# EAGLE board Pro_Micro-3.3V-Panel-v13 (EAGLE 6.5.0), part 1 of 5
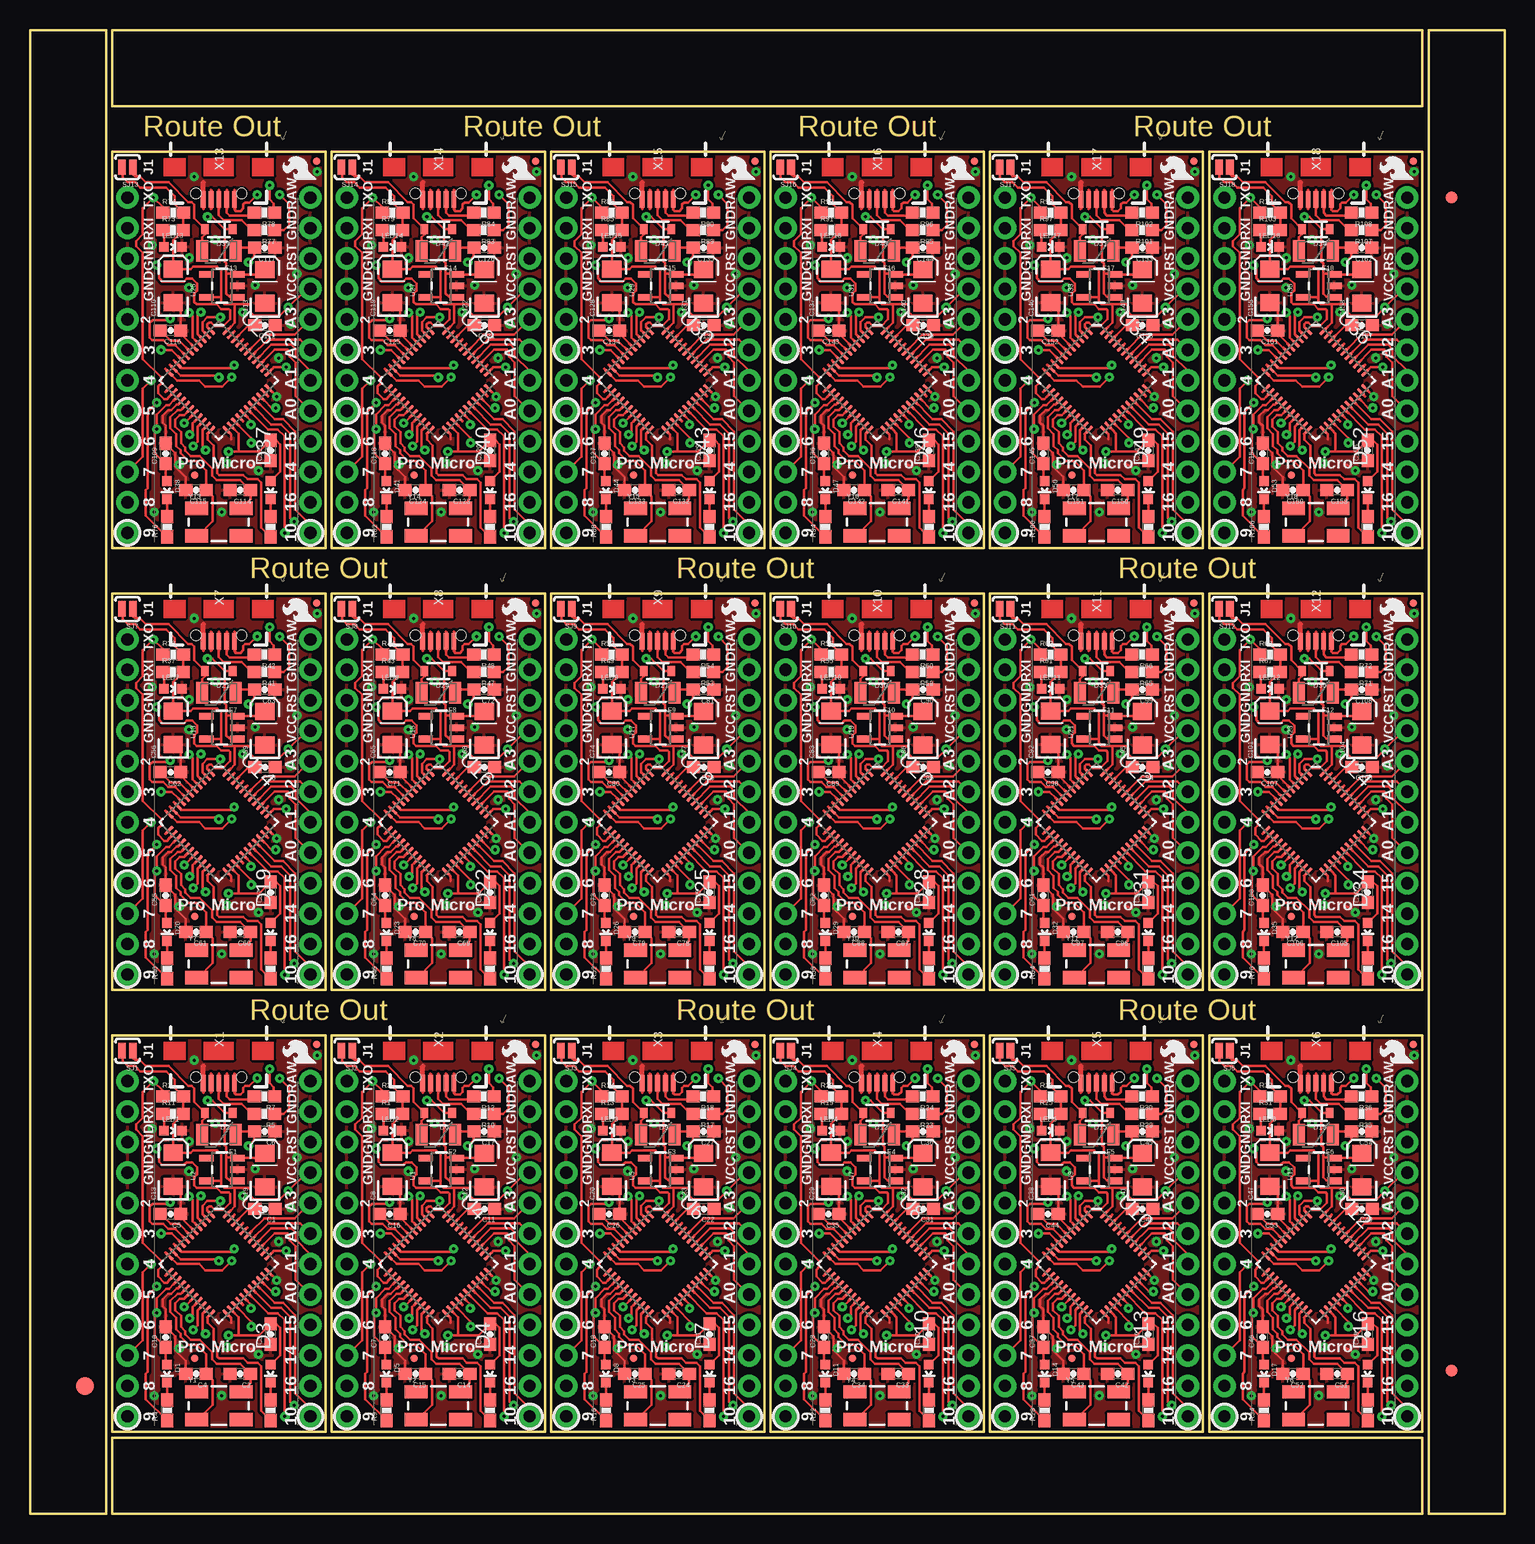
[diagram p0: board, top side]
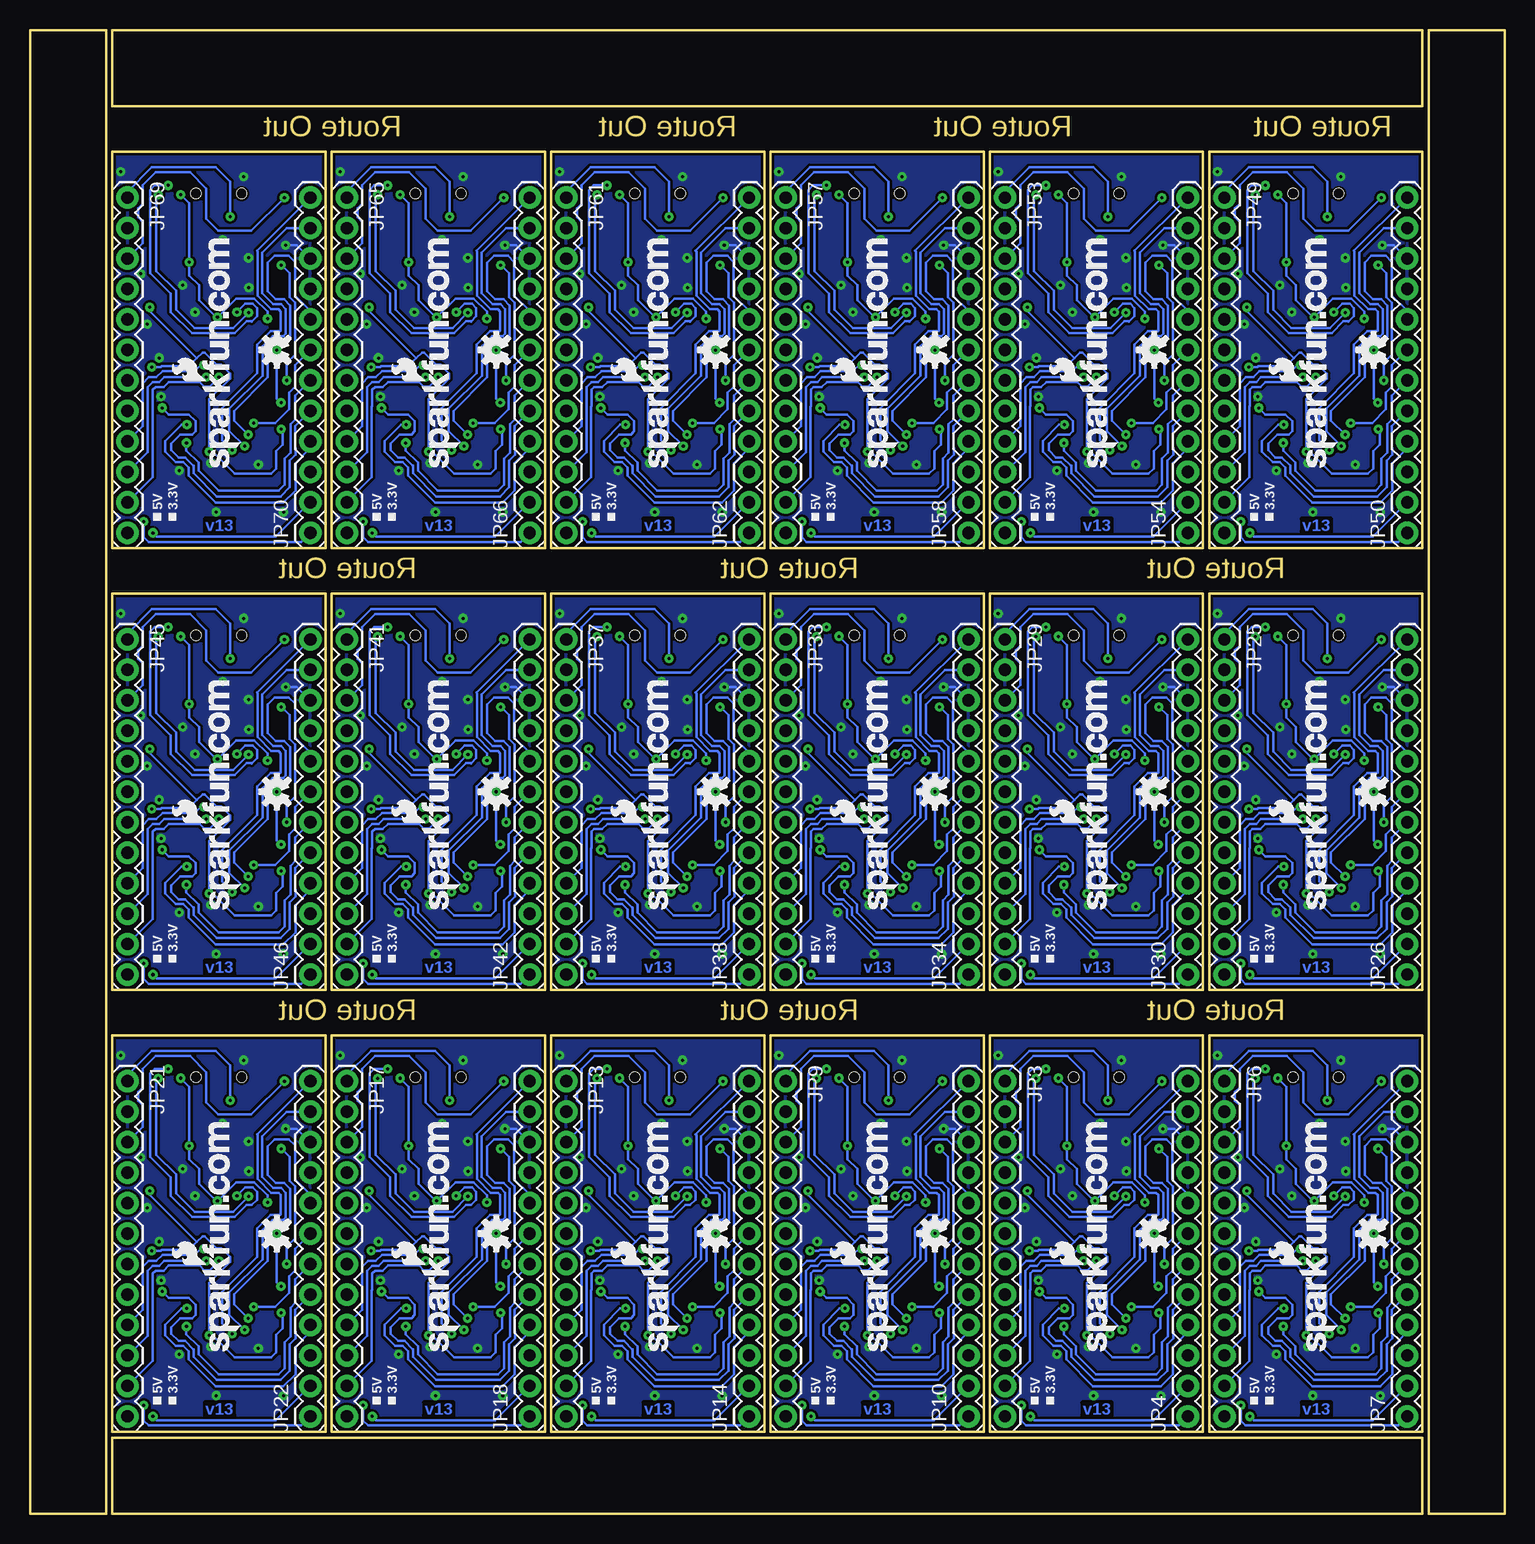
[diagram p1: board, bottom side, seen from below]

Size 122.94 x 123.7 mm. Coordinates in mm from the lower left corner, seen from the top.
Outline: 88 segments
Copper layers (1*16): Top 0.035mm / dielectric 1.5mm / Bottom 0.035mm
Design rules "SparkFun *": minimum track width 8mil, minimum drill 15mil, track to track 7mil, track to pad 7mil, pad to pad 7mil, via to via 7mil, smd to smd 7mil, copper to edge 7mil, drill to drill 7mil, minimum pad ring 12mil, minimum via ring 10mil, stop-mask expansion 4mil, vias tented up to drill 20mil, thermal gap 10mil
Net classes: 0 default: width 0.203 mm
tRestrict: area 16,16.4 to 16.2,16.6; area 19.9,20.4 to 20,20.5; area 12.3,17.1 to 19.4,24.4; area 34.3,16.4 to 34.5,16.6; area 38.2,20.4 to 38.3,20.5; area 30.6,17.1 to 37.7,24.4; area 52.6,16.4 to 52.8,16.6; area 56.5,20.4 to 56.6,20.5; area 48.9,17.1 to 56,24.4; area 70.9,16.4 to 71.1,16.6; area 74.8,20.4 to 74.9,20.5; area 67.2,17.1 to 74.3,24.4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

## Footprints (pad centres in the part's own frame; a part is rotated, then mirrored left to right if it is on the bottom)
0603-CAP = smd 1.1 x 1: 1 -0.85,0; 2 0.85,0
EIA3216 = smd 1.4 x 1.6: A 1.4,0; C -1.4,0
LED-0603 = smd 0.8 x 0.8: A 0,-0.75; C 0,0.75
SOD-323 = smd 0.63 x 0.83: 1 -1.15,0; 2 1.15,0
FIDUCIAL-1.5X3 = smd 1.5 x 1.5: 1 0,0
FIDUCIAL-1X2 = smd 1 x 1: 1 0,0
PTC-1206 = smd 1 x 1.8: 1 -1.4,0; 2 1.4,0
MICRO-FIDUCIAL = smd 0.635 x 0.635: 1 0,0
1X12 = drill 1.016 pad 1.88: 1 0,0; 2 2.54,0; 3 5.08,0; 4 7.62,0; 5 10.16,0; 6 12.7,0; 7 15.24,0; 8 17.78,0; 9 20.32,0; 10 22.86,0; 11 25.4,0; 12 27.94,0
0603-RES = smd 1.1 x 1: 1 -0.85,0; 2 0.85,0
SJ_2S-NO = smd 0.635 x 1.27: 1 -0.45,0; 2 0.45,0
SOT23-5 = smd 0.55 x 1.2: 1 -0.95,-1.3; 2 0,-1.3; 3 0.95,-1.3; 4 0.95,1.3; 5 -0.95,1.3
QFN-44-NOPAD_1:1-OUTFAKES = smd 0.8 x 0.3: 1 -3.337,2.465; 2 -3.337,1.972; 3 -3.337,1.479; 4 -3.337,0.986; 5 -3.337,0.493; 6 -3.337,0; 7 -3.337,-0.493; 8 -3.337,-0.986; 9 -3.337,-1.479; 10 -3.337,-1.972; 11 -3.337,-2.465; 23 3.337,-2.465; 24 3.337,-1.972; 25 3.337,-1.479; 26 3.337,-0.986; 27 3.337,-0.493; 28 3.337,0; 29 3.337,0.493; 30 3.337,0.986; 31 3.337,1.479; 32 3.337,1.972; 33 3.337,2.465 | smd 0.3 x 0.8: 12 -2.465,-3.337; 13 -1.972,-3.337; 14 -1.479,-3.337; 15 -0.986,-3.337; 16 -0.493,-3.337; 17 0,-3.337; 18 0.493,-3.337; 19 0.986,-3.337; 20 1.479,-3.337; 21 1.972,-3.337; 22 2.465,-3.337; 34 2.465,3.337; 35 1.972,3.337; 36 1.479,3.337; 37 0.986,3.337; 38 0.493,3.337; 39 0,3.337; 40 -0.493,3.337; 41 -0.986,3.337; 42 -1.479,3.337; 43 -1.972,3.337; 44 -2.465,3.337
USB-AB-MICRO-SMD-V03-IN&OUT = smd 1.4 x 0.4: D+1 2.7,0; D-1 2.7,0.65; GND1 2.7,-1.3; ID1 2.7,-0.65; VBUS1 2.7,1.3 | hole 0.85: 2.2,1.9; 2.2,-1.9
CRYSTAL-SMD-5X3 = smd 1.9 x 1.1: 1 -1.85,-1.15; 2 1.85,-1.15; 3 1.85,1.15; 4 -1.85,1.15

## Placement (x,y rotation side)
C1  0.1uF  [0603-CAP]  19.6,25.42 180 top
C2  22pF  [0603-CAP]  17.53,11.68 180 top
C3  0.1uF  [0603-CAP]  20.07,14.99 90 top
C4  22pF  [0603-CAP]  13.84,11.68 180 top
C5  1uF  [0603-CAP]  11.71,24.99 180 top
C6  1uF  [0603-CAP]  19.57,31.89 180 top
C7  1uF  [0603-CAP]  29.6,14.73 90 top
C8  10uF  [EIA3216]  30.21,28.71 90 top
C9  0.1uF  [0603-CAP]  38.35,14.99 90 top
C10  1uF  [0603-CAP]  11.32,14.73 90 top
C11  0.1uF  [0603-CAP]  37.88,25.42 180 top
C12  10uF  [EIA3216]  37.87,28.66 90 top
C13  10uF  [EIA3216]  11.93,28.71 90 top
C14  22pF  [0603-CAP]  35.81,11.68 180 top
C15  22pF  [0603-CAP]  32.13,11.68 180 top
C16  1uF  [0603-CAP]  30,24.99 180 top
C17  1uF  [0603-CAP]  37.86,31.89 180 top
C18  1uF  [0603-CAP]  47.89,14.73 90 top
C19  10uF  [EIA3216]  19.58,28.66 90 top
C20  10uF  [EIA3216]  48.5,28.71 90 top
C21  0.1uF  [0603-CAP]  56.64,14.99 90 top
C22  0.1uF  [0603-CAP]  56.17,25.42 180 top
C23  10uF  [EIA3216]  56.16,28.66 90 top
C24  22pF  [0603-CAP]  54.1,11.68 180 top
C25  22pF  [0603-CAP]  50.42,11.68 180 top
C26  1uF  [0603-CAP]  48.29,24.99 180 top
C27  1uF  [0603-CAP]  56.15,31.89 180 top
C28  1uF  [0603-CAP]  66.18,14.73 90 top
C29  10uF  [EIA3216]  66.79,28.71 90 top
C30  0.1uF  [0603-CAP]  74.93,14.99 90 top
C31  0.1uF  [0603-CAP]  74.46,25.42 180 top
C32  10uF  [EIA3216]  74.44,28.66 90 top
C33  22pF  [0603-CAP]  72.39,11.68 180 top
C34  22pF  [0603-CAP]  68.71,11.68 180 top
C35  1uF  [0603-CAP]  66.58,24.99 180 top
C36  1uF  [0603-CAP]  74.43,31.89 180 top
C37  1uF  [0603-CAP]  84.47,14.73 90 top
C38  10uF  [EIA3216]  85.08,28.71 90 top
C39  0.1uF  [0603-CAP]  93.22,14.99 90 top
C40  0.1uF  [0603-CAP]  92.75,25.42 180 top
C41  10uF  [EIA3216]  92.73,28.66 90 top
C42  22pF  [0603-CAP]  90.68,11.68 180 top
C43  22pF  [0603-CAP]  87,11.68 180 top
C44  1uF  [0603-CAP]  84.86,24.99 180 top
C45  1uF  [0603-CAP]  92.72,31.89 180 top
C46  1uF  [0603-CAP]  102.76,14.73 90 top
C47  10uF  [EIA3216]  103.37,28.71 90 top
C48  0.1uF  [0603-CAP]  111.51,14.99 90 top
C49  0.1uF  [0603-CAP]  111.04,25.42 180 top
C50  10uF  [EIA3216]  111.02,28.66 90 top
C51  22pF  [0603-CAP]  108.97,11.68 180 top
C52  22pF  [0603-CAP]  105.28,11.68 180 top
C53  1uF  [0603-CAP]  103.15,24.99 180 top
C54  1uF  [0603-CAP]  111.01,31.89 180 top
C55  1uF  [0603-CAP]  11.32,51.56 90 top
C56  10uF  [EIA3216]  11.93,65.54 90 top
C57  0.1uF  [0603-CAP]  20.07,51.82 90 top
C58  0.1uF  [0603-CAP]  19.6,62.25 180 top
C59  10uF  [EIA3216]  19.58,65.49 90 top
C60  22pF  [0603-CAP]  17.53,48.51 180 top
C61  22pF  [0603-CAP]  13.84,48.51 180 top
C62  1uF  [0603-CAP]  11.71,61.82 180 top
C63  1uF  [0603-CAP]  19.57,68.72 180 top
C64  1uF  [0603-CAP]  29.6,51.56 90 top
C65  10uF  [EIA3216]  30.21,65.54 90 top
C66  0.1uF  [0603-CAP]  38.35,51.82 90 top
C67  0.1uF  [0603-CAP]  37.88,62.25 180 top
C68  10uF  [EIA3216]  37.87,65.49 90 top
C69  22pF  [0603-CAP]  35.81,48.51 180 top
C70  22pF  [0603-CAP]  32.13,48.51 180 top
C71  1uF  [0603-CAP]  30,61.82 180 top
C72  1uF  [0603-CAP]  37.86,68.72 180 top
C73  1uF  [0603-CAP]  47.89,51.56 90 top
C74  10uF  [EIA3216]  48.5,65.54 90 top
C75  0.1uF  [0603-CAP]  56.64,51.82 90 top
C76  0.1uF  [0603-CAP]  56.17,62.25 180 top
C77  10uF  [EIA3216]  56.16,65.49 90 top
C78  22pF  [0603-CAP]  54.1,48.51 180 top
C79  22pF  [0603-CAP]  50.42,48.51 180 top
C80  1uF  [0603-CAP]  48.29,61.82 180 top
C81  1uF  [0603-CAP]  56.15,68.72 180 top
C82  1uF  [0603-CAP]  66.18,51.56 90 top
C83  10uF  [EIA3216]  66.79,65.54 90 top
C84  0.1uF  [0603-CAP]  74.93,51.82 90 top
C85  0.1uF  [0603-CAP]  74.46,62.25 180 top
C86  10uF  [EIA3216]  74.44,65.49 90 top
C87  22pF  [0603-CAP]  72.39,48.51 180 top
C88  22pF  [0603-CAP]  68.71,48.51 180 top
C89  1uF  [0603-CAP]  66.58,61.82 180 top
C90  1uF  [0603-CAP]  74.43,68.72 180 top
C91  1uF  [0603-CAP]  84.47,51.56 90 top
C92  10uF  [EIA3216]  85.08,65.54 90 top
C93  0.1uF  [0603-CAP]  93.22,51.82 90 top
C94  0.1uF  [0603-CAP]  92.75,62.25 180 top
C95  10uF  [EIA3216]  92.73,65.49 90 top
C96  22pF  [0603-CAP]  90.68,48.51 180 top
C97  22pF  [0603-CAP]  87,48.51 180 top
C98  1uF  [0603-CAP]  84.86,61.82 180 top
C99  1uF  [0603-CAP]  92.72,68.72 180 top
C100  1uF  [0603-CAP]  102.76,51.56 90 top
C101  10uF  [EIA3216]  103.37,65.54 90 top
C102  0.1uF  [0603-CAP]  111.51,51.82 90 top
C103  0.1uF  [0603-CAP]  111.04,62.25 180 top
C104  10uF  [EIA3216]  111.02,65.49 90 top
C105  22pF  [0603-CAP]  108.97,48.51 180 top
C106  22pF  [0603-CAP]  105.28,48.51 180 top
C107  1uF  [0603-CAP]  103.15,61.82 180 top
C108  1uF  [0603-CAP]  111.01,68.72 180 top
C109  1uF  [0603-CAP]  11.32,88.39 90 top
C110  10uF  [EIA3216]  11.93,102.37 90 top
C111  0.1uF  [0603-CAP]  20.07,88.65 90 top
C112  0.1uF  [0603-CAP]  19.6,99.08 180 top
C113  10uF  [EIA3216]  19.58,102.32 90 top
C114  22pF  [0603-CAP]  17.53,85.34 180 top
C115  22pF  [0603-CAP]  13.84,85.34 180 top
C116  1uF  [0603-CAP]  11.71,98.65 180 top
C117  1uF  [0603-CAP]  19.57,105.55 180 top
C118  1uF  [0603-CAP]  29.6,88.39 90 top
C119  10uF  [EIA3216]  30.21,102.37 90 top
C120  0.1uF  [0603-CAP]  38.35,88.65 90 top
C121  0.1uF  [0603-CAP]  37.88,99.08 180 top
C122  10uF  [EIA3216]  37.87,102.32 90 top
C123  22pF  [0603-CAP]  35.81,85.34 180 top
C124  22pF  [0603-CAP]  32.13,85.34 180 top
C125  1uF  [0603-CAP]  30,98.65 180 top
C126  1uF  [0603-CAP]  37.86,105.55 180 top
C127  1uF  [0603-CAP]  47.89,88.39 90 top
C128  10uF  [EIA3216]  48.5,102.37 90 top
C129  0.1uF  [0603-CAP]  56.64,88.65 90 top
C130  0.1uF  [0603-CAP]  56.17,99.08 180 top
C131  10uF  [EIA3216]  56.16,102.32 90 top
C132  22pF  [0603-CAP]  54.1,85.34 180 top
C133  22pF  [0603-CAP]  50.42,85.34 180 top
C134  1uF  [0603-CAP]  48.29,98.65 180 top
C135  1uF  [0603-CAP]  56.15,105.55 180 top
C136  1uF  [0603-CAP]  66.18,88.39 90 top
C137  10uF  [EIA3216]  66.79,102.37 90 top
C138  0.1uF  [0603-CAP]  74.93,88.65 90 top
C139  0.1uF  [0603-CAP]  74.46,99.08 180 top
C140  10uF  [EIA3216]  74.44,102.32 90 top
C141  22pF  [0603-CAP]  72.39,85.34 180 top
C142  22pF  [0603-CAP]  68.71,85.34 180 top
C143  1uF  [0603-CAP]  66.58,98.65 180 top
C144  1uF  [0603-CAP]  74.43,105.55 180 top
C145  1uF  [0603-CAP]  84.47,88.39 90 top
C146  10uF  [EIA3216]  85.08,102.37 90 top
C147  0.1uF  [0603-CAP]  93.22,88.65 90 top
C148  0.1uF  [0603-CAP]  92.75,99.08 180 top
C149  10uF  [EIA3216]  92.73,102.32 90 top
C150  22pF  [0603-CAP]  90.68,85.34 180 top
C151  22pF  [0603-CAP]  87,85.34 180 top
C152  1uF  [0603-CAP]  84.86,98.65 180 top
C153  1uF  [0603-CAP]  92.72,105.55 180 top
C154  1uF  [0603-CAP]  102.76,88.39 90 top
C155  10uF  [EIA3216]  103.37,102.37 90 top
C156  0.1uF  [0603-CAP]  111.51,88.65 90 top
C157  0.1uF  [0603-CAP]  111.04,99.08 180 top
C158  10uF  [EIA3216]  111.02,102.32 90 top
C159  22pF  [0603-CAP]  108.97,85.34 180 top
C160  22pF  [0603-CAP]  105.28,85.34 180 top
C161  1uF  [0603-CAP]  103.15,98.65 180 top
C162  1uF  [0603-CAP]  111.01,105.55 180 top
D1  Yellow  [LED-0603]  11.43,11.68 180 top
D2  [SOD-323]  15.75,33.43 180 top
D3  Green  [LED-0603]  20.07,11.68 180 top
D4  Green  [LED-0603]  38.35,11.68 180 top
D5  Yellow  [LED-0603]  29.72,11.68 180 top
D6  [SOD-323]  34.04,33.43 180 top
D7  Green  [LED-0603]  56.64,11.68 180 top
D8  Yellow  [LED-0603]  48.01,11.68 180 top
D9  [SOD-323]  52.32,33.43 180 top
D10  Green  [LED-0603]  74.93,11.68 180 top
D11  Yellow  [LED-0603]  66.29,11.68 180 top
D12  [SOD-323]  70.61,33.43 180 top
D13  Green  [LED-0603]  93.22,11.68 180 top
D14  Yellow  [LED-0603]  84.58,11.68 180 top
D15  [SOD-323]  88.9,33.43 180 top
D16  Green  [LED-0603]  111.51,11.68 180 top
D17  Yellow  [LED-0603]  102.87,11.68 180 top
D18  [SOD-323]  107.19,33.43 180 top
D19  Green  [LED-0603]  20.07,48.51 180 top
D20  Yellow  [LED-0603]  11.43,48.51 180 top
D21  [SOD-323]  15.75,70.26 180 top
D22  Green  [LED-0603]  38.35,48.51 180 top
D23  Yellow  [LED-0603]  29.72,48.51 180 top
D24  [SOD-323]  34.04,70.26 180 top
D25  Green  [LED-0603]  56.64,48.51 180 top
D26  Yellow  [LED-0603]  48.01,48.51 180 top
D27  [SOD-323]  52.32,70.26 180 top
D28  Green  [LED-0603]  74.93,48.51 180 top
D29  Yellow  [LED-0603]  66.29,48.51 180 top
D30  [SOD-323]  70.61,70.26 180 top
D31  Green  [LED-0603]  93.22,48.51 180 top
D32  Yellow  [LED-0603]  84.58,48.51 180 top
D33  [SOD-323]  88.9,70.26 180 top
D34  Green  [LED-0603]  111.51,48.51 180 top
D35  Yellow  [LED-0603]  102.87,48.51 180 top
D36  [SOD-323]  107.19,70.26 180 top
D37  Green  [LED-0603]  20.07,85.34 180 top
D38  Yellow  [LED-0603]  11.43,85.34 180 top
D39  [SOD-323]  15.75,107.09 180 top
D40  Green  [LED-0603]  38.35,85.34 180 top
D41  Yellow  [LED-0603]  29.72,85.34 180 top
D42  [SOD-323]  34.04,107.09 180 top
D43  Green  [LED-0603]  56.64,85.34 180 top
D44  Yellow  [LED-0603]  48.01,85.34 180 top
D45  [SOD-323]  52.32,107.09 180 top
D46  Green  [LED-0603]  74.93,85.34 180 top
D47  Yellow  [LED-0603]  66.29,85.34 180 top
D48  [SOD-323]  70.61,107.09 180 top
D49  Green  [LED-0603]  93.22,85.34 180 top
D50  Yellow  [LED-0603]  84.58,85.34 180 top
D51  [SOD-323]  88.9,107.09 180 top
D52  Green  [LED-0603]  111.51,85.34 180 top
D53  Yellow  [LED-0603]  102.87,85.34 180 top
D54  [SOD-323]  107.19,107.09 180 top
E$1  [FIDUCIAL-1.5X3]  4.57,10.67 0 top
E$4  [FIDUCIAL-1X2]  118.49,11.94 0 top
E$8  [FIDUCIAL-1X2]  118.49,109.73 180 top
F1  500mA  [PTC-1206]  15.75,31.62 180 top
F2  500mA  [PTC-1206]  34.04,31.62 180 top
F3  500mA  [PTC-1206]  52.32,31.62 180 top
F4  500mA  [PTC-1206]  70.61,31.62 180 top
F5  500mA  [PTC-1206]  88.9,31.62 180 top
F6  500mA  [PTC-1206]  107.19,31.62 180 top
F7  500mA  [PTC-1206]  15.75,68.45 180 top
F8  500mA  [PTC-1206]  34.04,68.45 180 top
F9  500mA  [PTC-1206]  52.32,68.45 180 top
F10  500mA  [PTC-1206]  70.61,68.45 180 top
F11  500mA  [PTC-1206]  88.9,68.45 180 top
F12  500mA  [PTC-1206]  107.19,68.45 180 top
F13  500mA  [PTC-1206]  15.75,105.28 180 top
F14  500mA  [PTC-1206]  34.04,105.28 180 top
F15  500mA  [PTC-1206]  52.32,105.28 180 top
F16  500mA  [PTC-1206]  70.61,105.28 180 top
F17  500mA  [PTC-1206]  88.9,105.28 180 top
F18  500mA  [PTC-1206]  107.19,105.28 180 top
JP1  FIDUCIALUFIDUCIAL  [MICRO-FIDUCIAL]  13.72,12.95 0 top
JP2  FIDUCIALUFIDUCIAL  [MICRO-FIDUCIAL]  23.88,39.12 0 top
JP3  [1X12]  41.66,36.07 270 bottom
JP4  [1X12]  26.42,8.13 90 bottom
JP5  FIDUCIALUFIDUCIAL  [MICRO-FIDUCIAL]  32,12.95 0 top
JP6  [1X12]  23.37,36.07 270 bottom
JP7  [1X12]  8.13,8.13 90 bottom
JP8  FIDUCIALUFIDUCIAL  [MICRO-FIDUCIAL]  42.16,39.12 0 top
JP9  [1X12]  59.94,36.07 270 bottom
JP10  [1X12]  44.7,8.13 90 bottom
JP11  FIDUCIALUFIDUCIAL  [MICRO-FIDUCIAL]  50.29,12.95 0 top
JP12  FIDUCIALUFIDUCIAL  [MICRO-FIDUCIAL]  60.45,39.12 0 top
JP13  [1X12]  78.23,36.07 270 bottom
JP14  [1X12]  62.99,8.13 90 bottom
JP15  FIDUCIALUFIDUCIAL  [MICRO-FIDUCIAL]  68.58,12.95 0 top
JP16  FIDUCIALUFIDUCIAL  [MICRO-FIDUCIAL]  78.74,39.12 0 top
JP17  [1X12]  96.52,36.07 270 bottom
JP18  [1X12]  81.28,8.13 90 bottom
JP19  FIDUCIALUFIDUCIAL  [MICRO-FIDUCIAL]  86.87,12.95 0 top
JP20  FIDUCIALUFIDUCIAL  [MICRO-FIDUCIAL]  97.03,39.12 0 top
JP21  [1X12]  114.81,36.07 270 bottom
JP22  [1X12]  99.57,8.13 90 bottom
JP23  FIDUCIALUFIDUCIAL  [MICRO-FIDUCIAL]  105.16,12.95 0 top
JP24  FIDUCIALUFIDUCIAL  [MICRO-FIDUCIAL]  115.32,39.12 0 top
JP25  [1X12]  23.37,72.9 270 bottom
JP26  [1X12]  8.13,44.96 90 bottom
JP27  FIDUCIALUFIDUCIAL  [MICRO-FIDUCIAL]  13.72,49.78 0 top
JP28  FIDUCIALUFIDUCIAL  [MICRO-FIDUCIAL]  23.88,75.95 0 top
JP29  [1X12]  41.66,72.9 270 bottom
JP30  [1X12]  26.42,44.96 90 bottom
JP31  FIDUCIALUFIDUCIAL  [MICRO-FIDUCIAL]  32,49.78 0 top
JP32  FIDUCIALUFIDUCIAL  [MICRO-FIDUCIAL]  42.16,75.95 0 top
JP33  [1X12]  59.94,72.9 270 bottom
JP34  [1X12]  44.7,44.96 90 bottom
JP35  FIDUCIALUFIDUCIAL  [MICRO-FIDUCIAL]  50.29,49.78 0 top
JP36  FIDUCIALUFIDUCIAL  [MICRO-FIDUCIAL]  60.45,75.95 0 top
JP37  [1X12]  78.23,72.9 270 bottom
JP38  [1X12]  62.99,44.96 90 bottom
JP39  FIDUCIALUFIDUCIAL  [MICRO-FIDUCIAL]  68.58,49.78 0 top
JP40  FIDUCIALUFIDUCIAL  [MICRO-FIDUCIAL]  78.74,75.95 0 top
JP41  [1X12]  96.52,72.9 270 bottom
JP42  [1X12]  81.28,44.96 90 bottom
JP43  FIDUCIALUFIDUCIAL  [MICRO-FIDUCIAL]  86.87,49.78 0 top
JP44  FIDUCIALUFIDUCIAL  [MICRO-FIDUCIAL]  97.03,75.95 0 top
JP45  [1X12]  114.81,72.9 270 bottom
JP46  [1X12]  99.57,44.96 90 bottom
JP47  FIDUCIALUFIDUCIAL  [MICRO-FIDUCIAL]  105.16,49.78 0 top
JP48  FIDUCIALUFIDUCIAL  [MICRO-FIDUCIAL]  115.32,75.95 0 top
JP49  [1X12]  23.37,109.73 270 bottom
JP50  [1X12]  8.13,81.79 90 bottom
JP51  FIDUCIALUFIDUCIAL  [MICRO-FIDUCIAL]  13.72,86.61 0 top
JP52  FIDUCIALUFIDUCIAL  [MICRO-FIDUCIAL]  23.88,112.78 0 top
JP53  [1X12]  41.66,109.73 270 bottom
JP54  [1X12]  26.42,81.79 90 bottom
JP55  FIDUCIALUFIDUCIAL  [MICRO-FIDUCIAL]  32,86.61 0 top
JP56  FIDUCIALUFIDUCIAL  [MICRO-FIDUCIAL]  42.16,112.78 0 top
JP57  [1X12]  59.94,109.73 270 bottom
JP58  [1X12]  44.7,81.79 90 bottom
JP59  FIDUCIALUFIDUCIAL  [MICRO-FIDUCIAL]  50.29,86.61 0 top
JP60  FIDUCIALUFIDUCIAL  [MICRO-FIDUCIAL]  60.45,112.78 0 top
JP61  [1X12]  78.23,109.73 270 bottom
JP62  [1X12]  62.99,81.79 90 bottom
JP63  FIDUCIALUFIDUCIAL  [MICRO-FIDUCIAL]  68.58,86.61 0 top
JP64  FIDUCIALUFIDUCIAL  [MICRO-FIDUCIAL]  78.74,112.78 0 top
JP65  [1X12]  96.52,109.73 270 bottom
JP66  [1X12]  81.28,81.79 90 bottom
JP67  FIDUCIALUFIDUCIAL  [MICRO-FIDUCIAL]  86.87,86.61 0 top
JP68  FIDUCIALUFIDUCIAL  [MICRO-FIDUCIAL]  97.03,112.78 0 top
JP69  [1X12]  114.81,109.73 270 bottom
JP70  [1X12]  99.57,81.79 90 bottom
JP71  FIDUCIALUFIDUCIAL  [MICRO-FIDUCIAL]  105.16,86.61 0 top
JP72  FIDUCIALUFIDUCIAL  [MICRO-FIDUCIAL]  115.32,112.78 0 top
LED1  Red  [LED-0603]  11.93,31.96 270 top
LED2  Red  [LED-0603]  30.21,31.96 270 top
LED3  Red  [LED-0603]  48.5,31.96 270 top
LED4  Red  [LED-0603]  66.79,31.96 270 top
LED5  Red  [LED-0603]  85.08,31.96 270 top
LED6  Red  [LED-0603]  103.37,31.96 270 top
LED7  Red  [LED-0603]  11.93,68.79 270 top
LED8  Red  [LED-0603]  30.21,68.79 270 top
LED9  Red  [LED-0603]  48.5,68.79 270 top
LED10  Red  [LED-0603]  66.79,68.79 270 top
LED11  Red  [LED-0603]  85.08,68.79 270 top
LED12  Red  [LED-0603]  103.37,68.79 270 top
LED13  Red  [LED-0603]  11.93,105.62 270 top
LED14  Red  [LED-0603]  30.21,105.62 270 top
LED15  Red  [LED-0603]  48.5,105.62 270 top
LED16  Red  [LED-0603]  66.79,105.62 270 top
LED17  Red  [LED-0603]  85.08,105.62 270 top
LED18  Red  [LED-0603]  103.37,105.62 270 top
R1  1K  [0603-RES]  30.21,33.36 0 top
R2  10K  [0603-RES]  11.94,34.8 0 top
R3  10K  [0603-RES]  30.23,34.8 0 top
R4  330  [0603-RES]  11.43,8.64 90 top
R5  22  [0603-RES]  19.56,33.35 180 top
R6  330  [0603-RES]  20.07,8.64 90 top
R7  22  [0603-RES]  19.56,34.8 180 top
R8  330  [0603-RES]  38.35,8.64 90 top
R9  330  [0603-RES]  29.72,8.64 90 top
R10  22  [0603-RES]  37.85,33.35 180 top
R11  1K  [0603-RES]  11.93,33.36 0 top
R12  22  [0603-RES]  37.85,34.8 180 top
R13  1K  [0603-RES]  48.5,33.36 0 top
R14  10K  [0603-RES]  48.51,34.8 0 top
R15  330  [0603-RES]  56.64,8.64 90 top
R16  330  [0603-RES]  48.01,8.64 90 top
R17  22  [0603-RES]  56.13,33.35 180 top
R18  22  [0603-RES]  56.13,34.8 180 top
R19  1K  [0603-RES]  66.79,33.36 0 top
R20  10K  [0603-RES]  66.8,34.8 0 top
R21  330  [0603-RES]  74.93,8.64 90 top
R22  330  [0603-RES]  66.29,8.64 90 top
R23  22  [0603-RES]  74.42,33.35 180 top
R24  22  [0603-RES]  74.42,34.8 180 top
R25  1K  [0603-RES]  85.08,33.36 0 top
R26  10K  [0603-RES]  85.09,34.8 0 top
R27  330  [0603-RES]  93.22,8.64 90 top
R28  330  [0603-RES]  84.58,8.64 90 top
R29  22  [0603-RES]  92.71,33.35 180 top
R30  22  [0603-RES]  92.71,34.8 180 top
R31  1K  [0603-RES]  103.37,33.36 0 top
R32  10K  [0603-RES]  103.38,34.8 0 top
R33  330  [0603-RES]  111.51,8.64 90 top
R34  330  [0603-RES]  102.87,8.64 90 top
R35  22  [0603-RES]  111,33.35 180 top
R36  22  [0603-RES]  111,34.8 180 top
R37  1K  [0603-RES]  11.93,70.19 0 top
R38  10K  [0603-RES]  11.94,71.63 0 top
R39  330  [0603-RES]  20.07,45.47 90 top
R40  330  [0603-RES]  11.43,45.47 90 top
R41  22  [0603-RES]  19.56,70.18 180 top
R42  22  [0603-RES]  19.56,71.63 180 top
R43  1K  [0603-RES]  30.21,70.19 0 top
R44  10K  [0603-RES]  30.23,71.63 0 top
R45  330  [0603-RES]  38.35,45.47 90 top
R46  330  [0603-RES]  29.72,45.47 90 top
R47  22  [0603-RES]  37.85,70.18 180 top
R48  22  [0603-RES]  37.85,71.63 180 top
R49  1K  [0603-RES]  48.5,70.19 0 top
R50  10K  [0603-RES]  48.51,71.63 0 top
R51  330  [0603-RES]  56.64,45.47 90 top
R52  330  [0603-RES]  48.01,45.47 90 top
R53  22  [0603-RES]  56.13,70.18 180 top
R54  22  [0603-RES]  56.13,71.63 180 top
R55  1K  [0603-RES]  66.79,70.19 0 top
R56  10K  [0603-RES]  66.8,71.63 0 top
R57  330  [0603-RES]  74.93,45.47 90 top
R58  330  [0603-RES]  66.29,45.47 90 top
R59  22  [0603-RES]  74.42,70.18 180 top
R60  22  [0603-RES]  74.42,71.63 180 top
R61  1K  [0603-RES]  85.08,70.19 0 top
R62  10K  [0603-RES]  85.09,71.63 0 top
R63  330  [0603-RES]  93.22,45.47 90 top
R64  330  [0603-RES]  84.58,45.47 90 top
R65  22  [0603-RES]  92.71,70.18 180 top
R66  22  [0603-RES]  92.71,71.63 180 top
R67  1K  [0603-RES]  103.37,70.19 0 top
R68  10K  [0603-RES]  103.38,71.63 0 top
R69  330  [0603-RES]  111.51,45.47 90 top
R70  330  [0603-RES]  102.87,45.47 90 top
R71  22  [0603-RES]  111,70.18 180 top
R72  22  [0603-RES]  111,71.63 180 top
R73  1K  [0603-RES]  11.93,107.02 0 top
R74  10K  [0603-RES]  11.94,108.46 0 top
R75  330  [0603-RES]  20.07,82.3 90 top
R76  330  [0603-RES]  11.43,82.3 90 top
R77  22  [0603-RES]  19.56,107.01 180 top
R78  22  [0603-RES]  19.56,108.46 180 top
R79  1K  [0603-RES]  30.21,107.02 0 top
R80  10K  [0603-RES]  30.23,108.46 0 top
R81  330  [0603-RES]  38.35,82.3 90 top
R82  330  [0603-RES]  29.72,82.3 90 top
R83  22  [0603-RES]  37.85,107.01 180 top
R84  22  [0603-RES]  37.85,108.46 180 top
R85  1K  [0603-RES]  48.5,107.02 0 top
R86  10K  [0603-RES]  48.51,108.46 0 top
R87  330  [0603-RES]  56.64,82.3 90 top
R88  330  [0603-RES]  48.01,82.3 90 top
R89  22  [0603-RES]  56.13,107.01 180 top
R90  22  [0603-RES]  56.13,108.46 180 top
R91  1K  [0603-RES]  66.79,107.02 0 top
R92  10K  [0603-RES]  66.8,108.46 0 top
R93  330  [0603-RES]  74.93,82.3 90 top
R94  330  [0603-RES]  66.29,82.3 90 top
R95  22  [0603-RES]  74.42,107.01 180 top
R96  22  [0603-RES]  74.42,108.46 180 top
R97  1K  [0603-RES]  85.08,107.02 0 top
R98  10K  [0603-RES]  85.09,108.46 0 top
R99  330  [0603-RES]  93.22,82.3 90 top
R100  330  [0603-RES]  84.58,82.3 90 top
R101  22  [0603-RES]  92.71,107.01 180 top
R102  22  [0603-RES]  92.71,108.46 180 top
R103  1K  [0603-RES]  103.37,107.02 0 top
R104  10K  [0603-RES]  103.38,108.46 0 top
R105  330  [0603-RES]  111.51,82.3 90 top
R106  330  [0603-RES]  102.87,82.3 90 top
R107  22  [0603-RES]  111,107.01 180 top
R108  22  [0603-RES]  111,108.46 180 top
SJ1  Closed for 5V Board  [SJ_2S-NO]  8.13,38.61 180 top
SJ2  Closed for 5V Board  [SJ_2S-NO]  26.42,38.61 180 top
SJ3  Closed for 5V Board  [SJ_2S-NO]  44.7,38.61 180 top
SJ4  Closed for 5V Board  [SJ_2S-NO]  62.99,38.61 180 top
SJ5  Closed for 5V Board  [SJ_2S-NO]  81.28,38.61 180 top
SJ6  Closed for 5V Board  [SJ_2S-NO]  99.57,38.61 180 top
SJ7  Closed for 5V Board  [SJ_2S-NO]  8.13,75.44 180 top
SJ8  Closed for 5V Board  [SJ_2S-NO]  26.42,75.44 180 top
SJ9  Closed for 5V Board  [SJ_2S-NO]  44.7,75.44 180 top
SJ10  Closed for 5V Board  [SJ_2S-NO]  62.99,75.44 180 top
SJ11  Closed for 5V Board  [SJ_2S-NO]  81.28,75.44 180 top
SJ12  Closed for 5V Board  [SJ_2S-NO]  99.57,75.44 180 top
SJ13  Closed for 5V Board  [SJ_2S-NO]  8.13,112.27 180 top
SJ14  Closed for 5V Board  [SJ_2S-NO]  26.42,112.27 180 top
SJ15  Closed for 5V Board  [SJ_2S-NO]  44.7,112.27 180 top
SJ16  Closed for 5V Board  [SJ_2S-NO]  62.99,112.27 180 top
SJ17  Closed for 5V Board  [SJ_2S-NO]  81.28,112.27 180 top
SJ18  Closed for 5V Board  [SJ_2S-NO]  99.57,112.27 180 top
U1  MIC5219  [SOT23-5]  34.28,28.71 90 top
U2  MIC5219  [SOT23-5]  15.99,28.71 90 top
U3  ATMEGA32U4  [QFN-44-NOPAD_1:1-OUTFAKES]  15.75,20.83 315 top
U4  ATMEGA32U4  [QFN-44-NOPAD_1:1-OUTFAKES]  34.04,20.83 315 top
U5  MIC5219  [SOT23-5]  52.57,28.71 90 top
U6  ATMEGA32U4  [QFN-44-NOPAD_1:1-OUTFAKES]  52.32,20.83 315 top
U7  MIC5219  [SOT23-5]  70.86,28.71 90 top
U8  ATMEGA32U4  [QFN-44-NOPAD_1:1-OUTFAKES]  70.61,20.83 315 top
U9  MIC5219  [SOT23-5]  89.15,28.71 90 top
U10  ATMEGA32U4  [QFN-44-NOPAD_1:1-OUTFAKES]  88.9,20.83 315 top
U11  MIC5219  [SOT23-5]  107.43,28.71 90 top
U12  ATMEGA32U4  [QFN-44-NOPAD_1:1-OUTFAKES]  107.19,20.83 315 top
U13  MIC5219  [SOT23-5]  15.99,65.54 90 top
U14  ATMEGA32U4  [QFN-44-NOPAD_1:1-OUTFAKES]  15.75,57.66 315 top
U15  MIC5219  [SOT23-5]  34.28,65.54 90 top
U16  ATMEGA32U4  [QFN-44-NOPAD_1:1-OUTFAKES]  34.04,57.66 315 top
U17  MIC5219  [SOT23-5]  52.57,65.54 90 top
U18  ATMEGA32U4  [QFN-44-NOPAD_1:1-OUTFAKES]  52.32,57.66 315 top
U19  MIC5219  [SOT23-5]  70.86,65.54 90 top
U20  ATMEGA32U4  [QFN-44-NOPAD_1:1-OUTFAKES]  70.61,57.66 315 top
U21  MIC5219  [SOT23-5]  89.15,65.54 90 top
U22  ATMEGA32U4  [QFN-44-NOPAD_1:1-OUTFAKES]  88.9,57.66 315 top
U23  MIC5219  [SOT23-5]  107.43,65.54 90 top
U24  ATMEGA32U4  [QFN-44-NOPAD_1:1-OUTFAKES]  107.19,57.66 315 top
U25  MIC5219  [SOT23-5]  15.99,102.37 90 top
U26  ATMEGA32U4  [QFN-44-NOPAD_1:1-OUTFAKES]  15.75,94.49 315 top
U27  MIC5219  [SOT23-5]  34.28,102.37 90 top
U28  ATMEGA32U4  [QFN-44-NOPAD_1:1-OUTFAKES]  34.04,94.49 315 top
U29  MIC5219  [SOT23-5]  52.57,102.37 90 top
U30  ATMEGA32U4  [QFN-44-NOPAD_1:1-OUTFAKES]  52.32,94.49 315 top
U31  MIC5219  [SOT23-5]  70.86,102.37 90 top
U32  ATMEGA32U4  [QFN-44-NOPAD_1:1-OUTFAKES]  70.61,94.49 315 top
U33  MIC5219  [SOT23-5]  89.15,102.37 90 top
U34  ATMEGA32U4  [QFN-44-NOPAD_1:1-OUTFAKES]  88.9,94.49 315 top
U35  MIC5219  [SOT23-5]  107.43,102.37 90 top
U36  ATMEGA32U4  [QFN-44-NOPAD_1:1-OUTFAKES]  107.19,94.49 315 top
U$1  LOGO-SFESK  [SFE-LOGO-FLAME]  23.88,37.59 90 top
U$2  LOGO-SFENEW  [SFE-NEW-WEBLOGO]  32.26,13.59 90 bottom
U$3  OSHW-LOGOS  [OSHW-LOGO-S]  10.92,23.37 90 bottom
U$4  LOGO-SFESK  [SFE-LOGO-FLAME]  42.16,37.59 90 top
U$5  OSHW-LOGOS  [OSHW-LOGO-S]  29.21,23.37 90 bottom
U$6  LOGO-SFENEW  [SFE-NEW-WEBLOGO]  50.55,13.59 90 bottom
U$7  LOGO-SFESK  [SFE-LOGO-FLAME]  60.45,37.59 90 top
U$8  OSHW-LOGOS  [OSHW-LOGO-S]  47.5,23.37 90 bottom
U$9  LOGO-SFENEW  [SFE-NEW-WEBLOGO]  68.83,13.59 90 bottom
U$10  LOGO-SFESK  [SFE-LOGO-FLAME]  78.74,37.59 90 top
U$11  LOGO-SFENEW  [SFE-NEW-WEBLOGO]  13.97,13.59 90 bottom
U$12  OSHW-LOGOS  [OSHW-LOGO-S]  65.79,23.37 90 bottom
U$13  LOGO-SFENEW  [SFE-NEW-WEBLOGO]  87.12,13.59 90 bottom
U$14  LOGO-SFESK  [SFE-LOGO-FLAME]  97.03,37.59 90 top
U$15  OSHW-LOGOS  [OSHW-LOGO-S]  84.07,23.37 90 bottom
U$16  LOGO-SFENEW  [SFE-NEW-WEBLOGO]  105.41,13.59 90 bottom
U$17  LOGO-SFESK  [SFE-LOGO-FLAME]  115.32,37.59 90 top
U$18  OSHW-LOGOS  [OSHW-LOGO-S]  102.36,23.37 90 bottom
U$19  LOGO-SFENEW  [SFE-NEW-WEBLOGO]  13.97,50.42 90 bottom
U$20  LOGO-SFESK  [SFE-LOGO-FLAME]  23.88,74.42 90 top
U$21  OSHW-LOGOS  [OSHW-LOGO-S]  10.92,60.2 90 bottom
U$22  LOGO-SFENEW  [SFE-NEW-WEBLOGO]  32.26,50.42 90 bottom
U$23  LOGO-SFESK  [SFE-LOGO-FLAME]  42.16,74.42 90 top
U$24  OSHW-LOGOS  [OSHW-LOGO-S]  29.21,60.2 90 bottom
U$25  LOGO-SFENEW  [SFE-NEW-WEBLOGO]  50.55,50.42 90 bottom
U$26  LOGO-SFESK  [SFE-LOGO-FLAME]  60.45,74.42 90 top
U$27  OSHW-LOGOS  [OSHW-LOGO-S]  47.5,60.2 90 bottom
U$28  LOGO-SFENEW  [SFE-NEW-WEBLOGO]  68.83,50.42 90 bottom
U$29  LOGO-SFESK  [SFE-LOGO-FLAME]  78.74,74.42 90 top
U$30  OSHW-LOGOS  [OSHW-LOGO-S]  65.79,60.2 90 bottom
U$31  LOGO-SFENEW  [SFE-NEW-WEBLOGO]  87.12,50.42 90 bottom
U$32  LOGO-SFESK  [SFE-LOGO-FLAME]  97.03,74.42 90 top
U$33  OSHW-LOGOS  [OSHW-LOGO-S]  84.07,60.2 90 bottom
U$34  LOGO-SFENEW  [SFE-NEW-WEBLOGO]  105.41,50.42 90 bottom
U$35  LOGO-SFESK  [SFE-LOGO-FLAME]  115.32,74.42 90 top
U$36  OSHW-LOGOS  [OSHW-LOGO-S]  102.36,60.2 90 bottom
U$37  LOGO-SFENEW  [SFE-NEW-WEBLOGO]  13.97,87.25 90 bottom
U$38  LOGO-SFESK  [SFE-LOGO-FLAME]  23.88,111.25 90 top
U$39  OSHW-LOGOS  [OSHW-LOGO-S]  10.92,97.03 90 bottom
U$40  LOGO-SFENEW  [SFE-NEW-WEBLOGO]  32.26,87.25 90 bottom
U$41  LOGO-SFESK  [SFE-LOGO-FLAME]  42.16,111.25 90 top
U$42  OSHW-LOGOS  [OSHW-LOGO-S]  29.21,97.03 90 bottom
U$43  LOGO-SFENEW  [SFE-NEW-WEBLOGO]  50.55,87.25 90 bottom
U$44  LOGO-SFESK  [SFE-LOGO-FLAME]  60.45,111.25 90 top
U$45  OSHW-LOGOS  [OSHW-LOGO-S]  47.5,97.03 90 bottom
U$46  LOGO-SFENEW  [SFE-NEW-WEBLOGO]  68.83,87.25 90 bottom
U$47  LOGO-SFESK  [SFE-LOGO-FLAME]  78.74,111.25 90 top
U$48  OSHW-LOGOS  [OSHW-LOGO-S]  65.79,97.03 90 bottom
U$49  LOGO-SFENEW  [SFE-NEW-WEBLOGO]  87.12,87.25 90 bottom
U$50  LOGO-SFESK  [SFE-LOGO-FLAME]  97.03,111.25 90 top
U$51  OSHW-LOGOS  [OSHW-LOGO-S]  84.07,97.03 90 bottom
U$52  LOGO-SFENEW  [SFE-NEW-WEBLOGO]  105.41,87.25 90 bottom
U$53  LOGO-SFESK  [SFE-LOGO-FLAME]  115.32,111.25 90 top
U$54  OSHW-LOGOS  [OSHW-LOGO-S]  102.36,97.03 90 bottom
X1  [USB-AB-MICRO-SMD-V03-IN&OUT]  15.75,38.61 270 top
X2  [USB-AB-MICRO-SMD-V03-IN&OUT]  34.04,38.61 270 top
X3  [USB-AB-MICRO-SMD-V03-IN&OUT]  52.32,38.61 270 top
X4  [USB-AB-MICRO-SMD-V03-IN&OUT]  70.61,38.61 270 top
X5  [USB-AB-MICRO-SMD-V03-IN&OUT]  88.9,38.61 270 top
X6  [USB-AB-MICRO-SMD-V03-IN&OUT]  107.19,38.61 270 top
X7  [USB-AB-MICRO-SMD-V03-IN&OUT]  15.75,75.44 270 top
X8  [USB-AB-MICRO-SMD-V03-IN&OUT]  34.04,75.44 270 top
X9  [USB-AB-MICRO-SMD-V03-IN&OUT]  52.32,75.44 270 top
X10  [USB-AB-MICRO-SMD-V03-IN&OUT]  70.61,75.44 270 top
X11  [USB-AB-MICRO-SMD-V03-IN&OUT]  88.9,75.44 270 top
X12  [USB-AB-MICRO-SMD-V03-IN&OUT]  107.19,75.44 270 top
X13  [USB-AB-MICRO-SMD-V03-IN&OUT]  15.75,112.27 270 top
X14  [USB-AB-MICRO-SMD-V03-IN&OUT]  34.04,112.27 270 top
X15  [USB-AB-MICRO-SMD-V03-IN&OUT]  52.32,112.27 270 top
X16  [USB-AB-MICRO-SMD-V03-IN&OUT]  70.61,112.27 270 top
X17  [USB-AB-MICRO-SMD-V03-IN&OUT]  88.9,112.27 270 top
X18  [USB-AB-MICRO-SMD-V03-IN&OUT]  107.19,112.27 270 top
Y1  16MHz  [CRYSTAL-SMD-5X3]  15.75,9.02 0 top
Y2  16MHz  [CRYSTAL-SMD-5X3]  34.04,9.02 0 top
Y3  16MHz  [CRYSTAL-SMD-5X3]  52.32,9.02 0 top
Y4  16MHz  [CRYSTAL-SMD-5X3]  70.61,9.02 0 top
Y5  16MHz  [CRYSTAL-SMD-5X3]  88.9,9.02 0 top
Y6  16MHz  [CRYSTAL-SMD-5X3]  107.19,9.02 0 top
Y7  16MHz  [CRYSTAL-SMD-5X3]  15.75,45.85 0 top
Y8  16MHz  [CRYSTAL-SMD-5X3]  34.04,45.85 0 top
Y9  16MHz  [CRYSTAL-SMD-5X3]  52.32,45.85 0 top
Y10  16MHz  [CRYSTAL-SMD-5X3]  70.61,45.85 0 top
Y11  16MHz  [CRYSTAL-SMD-5X3]  88.9,45.85 0 top
Y12  16MHz  [CRYSTAL-SMD-5X3]  107.19,45.85 0 top
Y13  16MHz  [CRYSTAL-SMD-5X3]  15.75,82.68 0 top
Y14  16MHz  [CRYSTAL-SMD-5X3]  34.04,82.68 0 top
Y15  16MHz  [CRYSTAL-SMD-5X3]  52.32,82.68 0 top
Y16  16MHz  [CRYSTAL-SMD-5X3]  70.61,82.68 0 top
Y17  16MHz  [CRYSTAL-SMD-5X3]  88.9,82.68 0 top
Y18  16MHz  [CRYSTAL-SMD-5X3]  107.19,82.68 0 top

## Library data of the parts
C1-C162 D1-D54 F1-F18 JP1-JP72 LED1-LED18 R1-R108 SJ1-SJ18 U1 U2 U5 U7 U9 U11 U13 U15 U17 U19 U21 U23 U25 U27 U29 U31 U33 U35 U$1-U$54 Y1-Y18 = SparkFun
E$1 E$4 E$8 = SparkFun-Aesthetics
U3 U4 U6 U8 U10 U12 U14 U16 U18 U20 U22 U24 U26 U28 U30 U32 U34 U36 X1-X18 = Testing

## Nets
A0: JP6.8 U3.36
A1: JP6.7 U3.37
A2: JP6.6 U3.38
A3: JP6.5 U3.39
A4: U3.40
A5: U3.41
A6: U4.41
A7: U4.40
A8: JP3.5 U4.39
A9: JP3.6 U4.38
A10: JP3.7 U4.37
A11: JP3.8 U4.36
A12: U6.41
A13: U6.40
A14: JP9.5 U6.39
A15: JP9.6 U6.38
A16: JP9.7 U6.37
A17: JP9.8 U6.36
A18: U8.41
A19: U8.40
A20: JP13.5 U8.39
A21: JP13.6 U8.38
A22: JP13.7 U8.37
A23: JP13.8 U8.36
A24: U10.41
A25: U10.40
A26: JP17.5 U10.39
A27: JP17.6 U10.38
A28: JP17.7 U10.37
A29: JP17.8 U10.36
A30: U12.41
A31: U12.40
A32: JP21.5 U12.39
A33: JP21.6 U12.38
A34: JP21.7 U12.37
A35: JP21.8 U12.36
A36: U14.41
A37: U14.40
A38: JP25.5 U14.39
A39: JP25.6 U14.38
A40: JP25.7 U14.37
A41: JP25.8 U14.36
A42: U16.41
A43: U16.40
A44: JP29.5 U16.39
A45: JP29.6 U16.38
A46: JP29.7 U16.37
A47: JP29.8 U16.36
A48: U18.41
A49: U18.40
A50: JP33.5 U18.39
A51: JP33.6 U18.38
A52: JP33.7 U18.37
A53: JP33.8 U18.36
A54: U20.41
A55: U20.40
A56: JP37.5 U20.39
A57: JP37.6 U20.38
A58: JP37.7 U20.37
A59: JP37.8 U20.36
A60: U22.41
A61: U22.40
A62: JP41.5 U22.39
A63: JP41.6 U22.38
A64: JP41.7 U22.37
A65: JP41.8 U22.36
A66: U24.41
A67: U24.40
A68: JP45.5 U24.39
A69: JP45.6 U24.38
A70: JP45.7 U24.37
A71: JP45.8 U24.36
A72: U26.41
A73: U26.40
A74: JP49.5 U26.39
A75: JP49.6 U26.38
A76: JP49.7 U26.37
A77: JP49.8 U26.36
A78: U28.41
A79: U28.40
A80: JP53.5 U28.39
A81: JP53.6 U28.38
A82: JP53.7 U28.37
A83: JP53.8 U28.36
A84: U30.41
A85: U30.40
A86: JP57.5 U30.39
A87: JP57.6 U30.38
A88: JP57.7 U30.37
A89: JP57.8 U30.36
A90: U32.41
A91: U32.40
A92: JP61.5 U32.39
A93: JP61.6 U32.38
A94: JP61.7 U32.37
A95: JP61.8 U32.36
A96: U34.41
A97: U34.40
A98: JP65.5 U34.39
A99: JP65.6 U34.38
A100: JP65.7 U34.37
A101: JP65.8 U34.36
A102: U36.41
A103: U36.40
A104: JP69.5 U36.39
A105: JP69.6 U36.38
A106: JP69.7 U36.37
A107: JP69.8 U36.36
AREF: C1.2 U3.42
AREF1: C11.2 U4.42
AREF2: C22.2 U6.42
AREF3: C31.2 U8.42
AREF4: C40.2 U10.42
AREF5: C49.2 U12.42
AREF6: C58.2 U14.42
AREF7: C67.2 U16.42
AREF8: C76.2 U18.42
AREF9: C85.2 U20.42
AREF10: C94.2 U22.42
AREF11: C103.2 U24.42
AREF12: C112.2 U26.42
AREF13: C121.2 U28.42
AREF14: C130.2 U30.42
AREF15: C139.2 U32.42
AREF16: C148.2 U34.42
AREF17: C157.2 U36.42
D1: JP4.1 U4.29
D2: JP7.8 U3.19
D3: JP7.7 U3.18
D4: JP7.6 U3.25
D5: JP7.5 U3.31
D6: JP7.4 U3.27
D7: JP7.3 U3.1
D8: JP7.2 U3.28
D9: JP7.1 U3.29
D10: JP6.12 U3.30
D11: U3.12
D12: U3.26
D13: U3.32
D14: R4.1 U3.8
D15: JP4.2 U4.28
D16: JP4.8 U4.19
D17: JP4.7 U4.18
D18: JP4.6 U4.25
D19: JP4.5 U4.31
D20: JP4.4 U4.27
D21: JP4.3 U4.1
D22: JP3.12 U4.30
D23: U4.12
D24: U4.26
D25: U4.32
D26: R9.1 U4.8
D27: JP10.1 U6.29
D28: JP10.2 U6.28
D29: JP10.8 U6.19
D30: JP10.7 U6.18
D31: JP10.6 U6.25
D32: JP10.5 U6.31
D33: JP10.4 U6.27
D34: JP10.3 U6.1
D35: JP9.12 U6.30
D36: U6.12
D37: U6.26
D38: U6.32
D39: R16.1 U6.8
D40: JP14.1 U8.29
D41: JP14.2 U8.28
D42: JP14.8 U8.19
D43: JP14.7 U8.18
D44: JP14.6 U8.25
D45: JP14.5 U8.31
D46: JP14.4 U8.27
D47: JP14.3 U8.1
D48: JP13.12 U8.30
D49: U8.12
D50: U8.26
D51: U8.32
D52: R22.1 U8.8
D53: JP18.1 U10.29
D54: JP18.2 U10.28
D55: JP18.8 U10.19
D56: JP18.7 U10.18
D57: JP18.6 U10.25
D58: JP18.5 U10.31
D59: JP18.4 U10.27
D60: JP18.3 U10.1
D61: JP17.12 U10.30
D62: U10.12
D63: U10.26
D64: U10.32
D65: R28.1 U10.8
D66: JP22.1 U12.29
D67: JP22.2 U12.28
D68: JP22.8 U12.19
D69: JP22.7 U12.18
D70: JP22.6 U12.25
D71: JP22.5 U12.31
D72: JP22.4 U12.27
D73: JP22.3 U12.1
D74: JP21.12 U12.30
D75: U12.12
D76: U12.26
D77: U12.32
D78: R34.1 U12.8
D79: JP26.1 U14.29
D80: JP26.2 U14.28
D81: JP26.8 U14.19
D82: JP26.7 U14.18
D83: JP26.6 U14.25
D84: JP26.5 U14.31
D85: JP26.4 U14.27
D86: JP26.3 U14.1
D87: JP25.12 U14.30
D88: U14.12
D89: U14.26
D90: U14.32
D91: R40.1 U14.8
D92: JP30.1 U16.29
D93: JP30.2 U16.28
D94: JP30.8 U16.19
D95: JP30.7 U16.18
D96: JP30.6 U16.25
D97: JP30.5 U16.31
D98: JP30.4 U16.27
D99: JP30.3 U16.1
D100: JP29.12 U16.30
D101: U16.12
D102: U16.26
D103: U16.32
D104: R46.1 U16.8
D105: JP34.1 U18.29
D106: JP34.2 U18.28
D107: JP34.8 U18.19
D108: JP34.7 U18.18
D109: JP34.6 U18.25
D110: JP34.5 U18.31
D111: JP34.4 U18.27
D112: JP34.3 U18.1
D113: JP33.12 U18.30
D114: U18.12
D115: U18.26
D116: U18.32
D117: R52.1 U18.8
D118: JP38.1 U20.29
D119: JP38.2 U20.28
D120: JP38.8 U20.19
D121: JP38.7 U20.18
D122: JP38.6 U20.25
D123: JP38.5 U20.31
D124: JP38.4 U20.27
D125: JP38.3 U20.1
D126: JP37.12 U20.30
D127: U20.12
D128: U20.26
D129: U20.32
D130: R58.1 U20.8
D131: JP42.1 U22.29
D132: JP42.2 U22.28
D133: JP42.8 U22.19
D134: JP42.7 U22.18
D135: JP42.6 U22.25
D136: JP42.5 U22.31
D137: JP42.4 U22.27
D138: JP42.3 U22.1
D139: JP41.12 U22.30
D140: U22.12
D141: U22.26
D142: U22.32
D143: R64.1 U22.8
D144: JP46.1 U24.29
D145: JP46.2 U24.28
D146: JP46.8 U24.19
D147: JP46.7 U24.18
D148: JP46.6 U24.25
D149: JP46.5 U24.31
D150: JP46.4 U24.27
D151: JP46.3 U24.1
D152: JP45.12 U24.30
D153: U24.12
D154: U24.26
D155: U24.32
D156: R70.1 U24.8
D157: JP50.1 U26.29
D158: JP50.2 U26.28
D159: JP50.8 U26.19
D160: JP50.7 U26.18
D161: JP50.6 U26.25
D162: JP50.5 U26.31
D163: JP50.4 U26.27
D164: JP50.3 U26.1
D165: JP49.12 U26.30
D166: U26.12
D167: U26.26
D168: U26.32
D169: R76.1 U26.8
D170: JP54.1 U28.29
D171: JP54.2 U28.28
D172: JP54.8 U28.19
D173: JP54.7 U28.18
D174: JP54.6 U28.25
D175: JP54.5 U28.31
D176: JP54.4 U28.27
D177: JP54.3 U28.1
D178: JP53.12 U28.30
D179: U28.12
D180: U28.26
D181: U28.32
D182: R82.1 U28.8
D183: JP58.1 U30.29
D184: JP58.2 U30.28
D185: JP58.8 U30.19
D186: JP58.7 U30.18
D187: JP58.6 U30.25
D188: JP58.5 U30.31
D189: JP58.4 U30.27
D190: JP58.3 U30.1
D191: JP57.12 U30.30
D192: U30.12
D193: U30.26
D194: U30.32
D195: R88.1 U30.8
D196: JP62.1 U32.29
D197: JP62.2 U32.28
D198: JP62.8 U32.19
D199: JP62.7 U32.18
D200: JP62.6 U32.25
D201: JP62.5 U32.31
D202: JP62.4 U32.27
D203: JP62.3 U32.1
D204: JP61.12 U32.30
D205: U32.12
D206: U32.26
D207: U32.32
D208: R94.1 U32.8
D209: JP66.1 U34.29
D210: JP66.2 U34.28
D211: JP66.8 U34.19
D212: JP66.7 U34.18
D213: JP66.6 U34.25
D214: JP66.5 U34.31
D215: JP66.4 U34.27
D216: JP66.3 U34.1
D217: JP65.12 U34.30
D218: U34.12
D219: U34.26
D220: U34.32
D221: R100.1 U34.8
D222: JP70.1 U36.29
D223: JP70.2 U36.28
D224: JP70.8 U36.19
D225: JP70.7 U36.18
D226: JP70.6 U36.25
D227: JP70.5 U36.31
D228: JP70.4 U36.27
D229: JP70.3 U36.1
D230: JP69.12 U36.30
D231: U36.12
D232: U36.26
D233: U36.32
D234: R106.1 U36.8
D+: R5.1 U3.4
D+1: R10.1 U4.4
D+2: R17.1 U6.4
D+3: R23.1 U8.4
D+4: R29.1 U10.4
D+5: R35.1 U12.4
D+6: R41.1 U14.4
D+7: R47.1 U16.4
D+8: R53.1 U18.4
D+9: R59.1 U20.4
D+10: R65.1 U22.4
D+11: R71.1 U24.4
D+12: R77.1 U26.4
D+13: R83.1 U28.4
D+14: R89.1 U30.4
D+15: R95.1 U32.4
D+16: R101.1 U34.4
D+17: R107.1 U36.4
D-: R7.1 U3.3
D-1: R12.1 U4.3
D-2: R18.1 U6.3
D-3: R24.1 U8.3
D-4: R30.1 U10.3
D-5: R36.1 U12.3
D-6: R42.1 U14.3
D-7: R48.1 U16.3
D-8: R54.1 U18.3
D-9: R60.1 U20.3
D-10: R66.1 U22.3
D-11: R72.1 U24.3
D-12: R78.1 U26.3
D-13: R84.1 U28.3
D-14: R90.1 U30.3
D-15: R96.1 U32.3
D-16: R102.1 U34.3
D-17: R108.1 U36.3
GND [vcc]: C1.1 C2.2 C3.1 C4.2 C5.1 C6.1 C10.2 C13.C C19.C JP6.2 JP7.9 JP7.10 LED1.C U2.2 U3.5 U3.15 U3.23 U3.33 U3.35 U3.43 X1.GND1
GND1 [vcc]: C7.2 C8.C C9.1 C11.1 C12.C C14.2 C15.2 C16.1 C17.1 JP3.2 JP4.9 JP4.10 LED2.C U1.2 U4.5 U4.15 U4.23 U4.33 U4.35 U4.43 X2.GND1
GND2 [vcc]: C18.2 C20.C C21.1 C22.1 C23.C C24.2 C25.2 C26.1 C27.1 JP9.2 JP10.9 JP10.10 LED3.C U5.2 U6.5 U6.15 U6.23 U6.33 U6.35 U6.43 X3.GND1
GND3 [vcc]: C28.2 C29.C C30.1 C31.1 C32.C C33.2 C34.2 C35.1 C36.1 JP13.2 JP14.9 JP14.10 LED4.C U7.2 U8.5 U8.15 U8.23 U8.33 U8.35 U8.43 X4.GND1
GND4 [vcc]: C37.2 C38.C C39.1 C40.1 C41.C C42.2 C43.2 C44.1 C45.1 JP17.2 JP18.9 JP18.10 LED5.C U9.2 U10.5 U10.15 U10.23 U10.33 U10.35 U10.43 X5.GND1
GND5 [vcc]: C46.2 C47.C C48.1 C49.1 C50.C C51.2 C52.2 C53.1 C54.1 JP21.2 JP22.9 JP22.10 LED6.C U11.2 U12.5 U12.15 U12.23 U12.33 U12.35 U12.43 X6.GND1
GND6 [vcc]: C55.2 C56.C C57.1 C58.1 C59.C C60.2 C61.2 C62.1 C63.1 JP25.2 JP26.9 JP26.10 LED7.C U13.2 U14.5 U14.15 U14.23 U14.33 U14.35 U14.43 X7.GND1
GND7 [vcc]: C64.2 C65.C C66.1 C67.1 C68.C C69.2 C70.2 C71.1 C72.1 JP29.2 JP30.9 JP30.10 LED8.C U15.2 U16.5 U16.15 U16.23 U16.33 U16.35 U16.43 X8.GND1
GND8 [vcc]: C73.2 C74.C C75.1 C76.1 C77.C C78.2 C79.2 C80.1 C81.1 JP33.2 JP34.9 JP34.10 LED9.C U17.2 U18.5 U18.15 U18.23 U18.33 U18.35 U18.43 X9.GND1
GND9 [vcc]: C82.2 C83.C C84.1 C85.1 C86.C C87.2 C88.2 C89.1 C90.1 JP37.2 JP38.9 JP38.10 LED10.C U19.2 U20.5 U20.15 U20.23 U20.33 U20.35 U20.43 X10.GND1
GND10 [vcc]: C91.2 C92.C C93.1 C94.1 C95.C C96.2 C97.2 C98.1 C99.1 JP41.2 JP42.9 JP42.10 LED11.C U21.2 U22.5 U22.15 U22.23 U22.33 U22.35 U22.43 X11.GND1
GND11 [vcc]: C100.2 C101.C C102.1 C103.1 C104.C C105.2 C106.2 C107.1 C108.1 JP45.2 JP46.9 JP46.10 LED12.C U23.2 U24.5 U24.15 U24.23 U24.33 U24.35 U24.43 X12.GND1
GND12 [vcc]: C109.2 C110.C C111.1 C112.1 C113.C C114.2 C115.2 C116.1 C117.1 JP49.2 JP50.9 JP50.10 LED13.C U25.2 U26.5 U26.15 U26.23 U26.33 U26.35 U26.43 X13.GND1
GND13 [vcc]: C118.2 C119.C C120.1 C121.1 C122.C C123.2 C124.2 C125.1 C126.1 JP53.2 JP54.9 JP54.10 LED14.C U27.2 U28.5 U28.15 U28.23 U28.33 U28.35 U28.43 X14.GND1
GND14 [vcc]: C127.2 C128.C C129.1 C130.1 C131.C C132.2 C133.2 C134.1 C135.1 JP57.2 JP58.9 JP58.10 LED15.C U29.2 U30.5 U30.15 U30.23 U30.33 U30.35 U30.43 X15.GND1
GND15 [vcc]: C136.2 C137.C C138.1 C139.1 C140.C C141.2 C142.2 C143.1 C144.1 JP61.2 JP62.9 JP62.10 LED16.C U31.2 U32.5 U32.15 U32.23 U32.33 U32.35 U32.43 X16.GND1
GND16 [vcc]: C145.2 C146.C C147.1 C148.1 C149.C C150.2 C151.2 C152.1 C153.1 JP65.2 JP66.9 JP66.10 LED17.C U33.2 U34.5 U34.15 U34.23 U34.33 U34.35 U34.43 X17.GND1
GND17 [vcc]: C154.2 C155.C C156.1 C157.1 C158.C C159.2 C160.2 C161.1 C162.1 JP69.2 JP70.9 JP70.10 LED18.C U35.2 U36.5 U36.15 U36.23 U36.33 U36.35 U36.43 X18.GND1
MISO: JP6.10 U3.11
MISO1: JP3.10 U4.11
MISO2: JP9.10 U6.11
MISO3: JP13.10 U8.11
MISO4: JP17.10 U10.11
MISO5: JP21.10 U12.11
MISO6: JP25.10 U14.11
MISO7: JP29.10 U16.11
MISO8: JP33.10 U18.11
MISO9: JP37.10 U20.11
MISO10: JP41.10 U22.11
MISO11: JP45.10 U24.11
MISO12: JP49.10 U26.11
MISO13: JP53.10 U28.11
MISO14: JP57.10 U30.11
MISO15: JP61.10 U32.11
MISO16: JP65.10 U34.11
MISO17: JP69.10 U36.11
MOSI: JP6.11 U3.10
MOSI1: JP3.11 U4.10
MOSI2: JP9.11 U6.10
MOSI3: JP13.11 U8.10
MOSI4: JP17.11 U10.10
MOSI5: JP21.11 U12.10
MOSI6: JP25.11 U14.10
MOSI7: JP29.11 U16.10
MOSI8: JP33.11 U18.10
MOSI9: JP37.11 U20.10
MOSI10: JP41.11 U22.10
MOSI11: JP45.11 U24.10
MOSI12: JP49.11 U26.10
MOSI13: JP53.11 U28.10
MOSI14: JP57.11 U30.10
MOSI15: JP61.11 U32.10
MOSI16: JP65.11 U34.10
MOSI17: JP69.11 U36.10
N$1: C4.1 U3.16 Y1.1
N$2: C2.1 U3.17 Y1.3
N$3: D2.2 F1.2 SJ1.1
N$4: C5.2 U3.6
N$5: D1.C R4.2
N$6: R7.2 X1.D-1
N$7: D3.C R6.2
N$8: R5.2 X1.D+1
N$9: LED2.A R1.1
N$10: C15.1 U4.16 Y2.1
N$11: C14.1 U4.17 Y2.3
N$12: C16.2 U4.6
N$13: R12.2 X2.D-1
N$14: R10.2 X2.D+1
N$15: D6.2 F2.2 SJ2.1
N$16: D5.C R9.2
N$17: D4.C R8.2
N$18: LED3.A R13.1
N$19: C25.1 U6.16 Y3.1
N$20: C24.1 U6.17 Y3.3
N$21: C26.2 U6.6
N$22: R18.2 X3.D-1
N$23: R17.2 X3.D+1
N$24: D9.2 F3.2 SJ3.1
N$25: D8.C R16.2
N$26: D7.C R15.2
N$27: LED4.A R19.1
N$28: C34.1 U8.16 Y4.1
N$29: C33.1 U8.17 Y4.3
N$30: C35.2 U8.6
N$31: R24.2 X4.D-1
N$32: R23.2 X4.D+1
N$33: D12.2 F4.2 SJ4.1
N$34: D11.C R22.2
N$35: D10.C R21.2
N$36: LED5.A R25.1
N$37: C43.1 U10.16 Y5.1
N$38: LED1.A R11.1
N$39: C42.1 U10.17 Y5.3
N$40: C44.2 U10.6
N$41: R30.2 X5.D-1
N$42: R29.2 X5.D+1
N$43: D15.2 F5.2 SJ5.1
N$44: D14.C R28.2
N$45: D13.C R27.2
N$46: LED6.A R31.1
N$47: C52.1 U12.16 Y6.1
N$48: C51.1 U12.17 Y6.3
N$49: C53.2 U12.6
N$50: R36.2 X6.D-1
N$51: R35.2 X6.D+1
N$52: D18.2 F6.2 SJ6.1
N$53: D17.C R34.2
N$54: D16.C R33.2
N$55: LED7.A R37.1
N$56: C61.1 U14.16 Y7.1
N$57: C60.1 U14.17 Y7.3
N$58: C62.2 U14.6
N$59: R42.2 X7.D-1
N$60: R41.2 X7.D+1
N$61: D21.2 F7.2 SJ7.1
N$62: D20.C R40.2
N$63: D19.C R39.2
N$64: LED8.A R43.1
N$65: C70.1 U16.16 Y8.1
N$66: C69.1 U16.17 Y8.3
N$67: C71.2 U16.6
N$68: R48.2 X8.D-1
N$69: R47.2 X8.D+1
N$70: D24.2 F8.2 SJ8.1
N$71: D23.C R46.2
N$72: D22.C R45.2
N$73: LED9.A R49.1
N$74: C79.1 U18.16 Y9.1
N$75: C78.1 U18.17 Y9.3
N$76: C80.2 U18.6
N$77: R54.2 X9.D-1
N$78: R53.2 X9.D+1
N$79: D27.2 F9.2 SJ9.1
N$80: D26.C R52.2
N$81: D25.C R51.2
N$82: LED10.A R55.1
N$83: C88.1 U20.16 Y10.1
N$84: C87.1 U20.17 Y10.3
N$85: C89.2 U20.6
N$86: R60.2 X10.D-1
N$87: R59.2 X10.D+1
N$88: D30.2 F10.2 SJ10.1
N$89: D29.C R58.2
N$90: D28.C R57.2
N$91: LED11.A R61.1
N$92: C97.1 U22.16 Y11.1
N$93: C96.1 U22.17 Y11.3
N$94: C98.2 U22.6
N$95: R66.2 X11.D-1
N$96: R65.2 X11.D+1
N$97: D33.2 F11.2 SJ11.1
N$98: D32.C R64.2
N$99: D31.C R63.2
N$100: LED12.A R67.1
N$101: C106.1 U24.16 Y12.1
N$102: C105.1 U24.17 Y12.3
N$103: C107.2 U24.6
N$104: R72.2 X12.D-1
N$105: R71.2 X12.D+1
N$106: D36.2 F12.2 SJ12.1
N$107: D35.C R70.2
N$108: D34.C R69.2
N$109: LED13.A R73.1
N$110: C115.1 U26.16 Y13.1
N$111: C114.1 U26.17 Y13.3
N$112: C116.2 U26.6
N$113: R78.2 X13.D-1
N$114: R77.2 X13.D+1
N$115: D39.2 F13.2 SJ13.1
N$116: D38.C R76.2
N$117: D37.C R75.2
N$118: LED14.A R79.1
N$119: C124.1 U28.16 Y14.1
N$120: C123.1 U28.17 Y14.3
N$121: C125.2 U28.6
N$122: R84.2 X14.D-1
N$123: R83.2 X14.D+1
N$124: D42.2 F14.2 SJ14.1
N$125: D41.C R82.2
N$126: D40.C R81.2
N$127: LED15.A R85.1
N$128: C133.1 U30.16 Y15.1
N$129: C132.1 U30.17 Y15.3
N$130: C134.2 U30.6
N$131: R90.2 X15.D-1
N$132: R89.2 X15.D+1
N$133: D45.2 F15.2 SJ15.1
N$134: D44.C R88.2
N$135: D43.C R87.2
N$136: LED16.A R91.1
N$137: C142.1 U32.16 Y16.1
N$138: C141.1 U32.17 Y16.3
N$139: C143.2 U32.6
N$140: R96.2 X16.D-1
N$141: R95.2 X16.D+1
N$142: D48.2 F16.2 SJ16.1
N$143: D47.C R94.2
N$144: D46.C R93.2
N$145: LED17.A R97.1
N$146: C151.1 U34.16 Y17.1
N$147: C150.1 U34.17 Y17.3
N$148: C152.2 U34.6
N$149: R102.2 X17.D-1
N$150: R101.2 X17.D+1
N$151: D51.2 F17.2 SJ17.1
N$152: D50.C R100.2
N$153: D49.C R99.2
N$154: LED18.A R103.1
N$155: C160.1 U36.16 Y18.1
N$156: C159.1 U36.17 Y18.3
N$157: C161.2 U36.6
N$158: R108.2 X18.D-1
N$159: R107.2 X18.D+1
N$160: D54.2 F18.2 SJ18.1
N$161: D53.C R106.2
N$162: D52.C R105.2
RAW [vcc]: C19.A D2.1 JP6.1 U2.1 U2.3
RAW1 [vcc]: C12.A D6.1 JP3.1 U1.1 U1.3
RAW2 [vcc]: C23.A D9.1 JP9.1 U5.1 U5.3
RAW3 [vcc]: C32.A D12.1 JP13.1 U7.1 U7.3
RAW4 [vcc]: C41.A D15.1 JP17.1 U9.1 U9.3
RAW5 [vcc]: C50.A D18.1 JP21.1 U11.1 U11.3
RAW6 [vcc]: C59.A D21.1 JP25.1 U13.1 U13.3
RAW7 [vcc]: C68.A D24.1 JP29.1 U15.1 U15.3
RAW8 [vcc]: C77.A D27.1 JP33.1 U17.1 U17.3
RAW9 [vcc]: C86.A D30.1 JP37.1 U19.1 U19.3
RAW10 [vcc]: C95.A D33.1 JP41.1 U21.1 U21.3
RAW11 [vcc]: C104.A D36.1 JP45.1 U23.1 U23.3
RAW12 [vcc]: C113.A D39.1 JP49.1 U25.1 U25.3
RAW13 [vcc]: C122.A D42.1 JP53.1 U27.1 U27.3
RAW14 [vcc]: C131.A D45.1 JP57.1 U29.1 U29.3
RAW15 [vcc]: C140.A D48.1 JP61.1 U31.1 U31.3
RAW16 [vcc]: C149.A D51.1 JP65.1 U33.1 U33.3
RAW17 [vcc]: C158.A D54.1 JP69.1 U35.1 U35.3
RESET: JP6.3 R2.1 U3.13
RESET1: JP3.3 R3.1 U4.13
RESET2: JP9.3 R14.1 U6.13
RESET3: JP13.3 R20.1 U8.13
RESET4: JP17.3 R26.1 U10.13
RESET5: JP21.3 R32.1 U12.13
RESET6: JP25.3 R38.1 U14.13
RESET7: JP29.3 R44.1 U16.13
RESET8: JP33.3 R50.1 U18.13
RESET9: JP37.3 R56.1 U20.13
RESET10: JP41.3 R62.1 U22.13
RESET11: JP45.3 R68.1 U24.13
RESET12: JP49.3 R74.1 U26.13
RESET13: JP53.3 R80.1 U28.13
RESET14: JP57.3 R86.1 U30.13
RESET15: JP61.3 R92.1 U32.13
RESET16: JP65.3 R98.1 U34.13
RESET17: JP69.3 R104.1 U36.13
RXI: JP7.11 U3.20
RXI1: JP4.11 U4.20
RXI2: JP10.11 U6.20
RXI3: JP14.11 U8.20
RXI4: JP18.11 U10.20
RXI5: JP22.11 U12.20
RXI6: JP26.11 U14.20
RXI7: JP30.11 U16.20
RXI8: JP34.11 U18.20
RXI9: JP38.11 U20.20
RXI10: JP42.11 U22.20
RXI11: JP46.11 U24.20
RXI12: JP50.11 U26.20
RXI13: JP54.11 U28.20
RXI14: JP58.11 U30.20
RXI15: JP62.11 U32.20
RXI16: JP66.11 U34.20
RXI17: JP70.11 U36.20
SCK: JP6.9 U3.9
SCK1: JP3.9 U4.9
SCK2: JP9.9 U6.9
SCK3: JP13.9 U8.9
SCK4: JP17.9 U10.9
SCK5: JP21.9 U12.9
SCK6: JP25.9 U14.9
SCK7: JP29.9 U16.9
SCK8: JP33.9 U18.9
SCK9: JP37.9 U20.9
SCK10: JP41.9 U22.9
SCK11: JP45.9 U24.9
SCK12: JP49.9 U26.9
SCK13: JP53.9 U28.9
SCK14: JP57.9 U30.9
SCK15: JP61.9 U32.9
SCK16: JP65.9 U34.9
SCK17: JP69.9 U36.9
TXLED: R6.1 U3.22
TXLED1: R8.1 U4.22
TXLED2: R15.1 U6.22
TXLED3: R21.1 U8.22
TXLED4: R27.1 U10.22
TXLED5: R33.1 U12.22
TXLED6: R39.1 U14.22
TXLED7: R45.1 U16.22
TXLED8: R51.1 U18.22
TXLED9: R57.1 U20.22
TXLED10: R63.1 U22.22
TXLED11: R69.1 U24.22
TXLED12: R75.1 U26.22
TXLED13: R81.1 U28.22
TXLED14: R87.1 U30.22
TXLED15: R93.1 U32.22
TXLED16: R99.1 U34.22
TXLED17: R105.1 U36.22
TXO: JP7.12 U3.21
TXO1: JP4.12 U4.21
TXO2: JP10.12 U6.21
TXO3: JP14.12 U8.21
TXO4: JP18.12 U10.21
TXO5: JP22.12 U12.21
TXO6: JP26.12 U14.21
TXO7: JP30.12 U16.21
TXO8: JP34.12 U18.21
TXO9: JP38.12 U20.21
TXO10: JP42.12 U22.21
TXO11: JP46.12 U24.21
TXO12: JP50.12 U26.21
TXO13: JP54.12 U28.21
TXO14: JP58.12 U30.21
TXO15: JP62.12 U32.21
TXO16: JP66.12 U34.21
TXO17: JP70.12 U36.21
UVCC: C6.2 F1.1 U3.2 U3.7 X1.VBUS1
UVCC1: C17.2 F2.1 U4.2 U4.7 X2.VBUS1
UVCC2: C27.2 F3.1 U6.2 U6.7 X3.VBUS1
UVCC3: C36.2 F4.1 U8.2 U8.7 X4.VBUS1
UVCC4: C45.2 F5.1 U10.2 U10.7 X5.VBUS1
UVCC5: C54.2 F6.1 U12.2 U12.7 X6.VBUS1
UVCC6: C63.2 F7.1 U14.2 U14.7 X7.VBUS1
UVCC7: C72.2 F8.1 U16.2 U16.7 X8.VBUS1
UVCC8: C81.2 F9.1 U18.2 U18.7 X9.VBUS1
UVCC9: C90.2 F10.1 U20.2 U20.7 X10.VBUS1
UVCC10: C99.2 F11.1 U22.2 U22.7 X11.VBUS1
UVCC11: C108.2 F12.1 U24.2 U24.7 X12.VBUS1
UVCC12: C117.2 F13.1 U26.2 U26.7 X13.VBUS1
UVCC13: C126.2 F14.1 U28.2 U28.7 X14.VBUS1
UVCC14: C135.2 F15.1 U30.2 U30.7 X15.VBUS1
UVCC15: C144.2 F16.1 U32.2 U32.7 X16.VBUS1
UVCC16: C153.2 F17.1 U34.2 U34.7 X17.VBUS1
UVCC17: C162.2 F18.1 U36.2 U36.7 X18.VBUS1
VCC: C3.2 C10.1 C13.A D1.A D3.A JP6.4 R2.2 R11.2 SJ1.2 U2.5 U3.14 U3.24 U3.34 U3.44
VCC1: C7.1 C8.A C9.2 D4.A D5.A JP3.4 R1.2 R3.2 SJ2.2 U1.5 U4.14 U4.24 U4.34 U4.44
VCC2: C18.1 C20.A C21.2 D7.A D8.A JP9.4 R13.2 R14.2 SJ3.2 U5.5 U6.14 U6.24 U6.34 U6.44
VCC3: C28.1 C29.A C30.2 D10.A D11.A JP13.4 R19.2 R20.2 SJ4.2 U7.5 U8.14 U8.24 U8.34 U8.44
VCC4: C37.1 C38.A C39.2 D13.A D14.A JP17.4 R25.2 R26.2 SJ5.2 U9.5 U10.14 U10.24 U10.34 U10.44
VCC5: C46.1 C47.A C48.2 D16.A D17.A JP21.4 R31.2 R32.2 SJ6.2 U11.5 U12.14 U12.24 U12.34 U12.44
VCC6: C55.1 C56.A C57.2 D19.A D20.A JP25.4 R37.2 R38.2 SJ7.2 U13.5 U14.14 U14.24 U14.34 U14.44
VCC7: C64.1 C65.A C66.2 D22.A D23.A JP29.4 R43.2 R44.2 SJ8.2 U15.5 U16.14 U16.24 U16.34 U16.44
VCC8: C73.1 C74.A C75.2 D25.A D26.A JP33.4 R49.2 R50.2 SJ9.2 U17.5 U18.14 U18.24 U18.34 U18.44
VCC9: C82.1 C83.A C84.2 D28.A D29.A JP37.4 R55.2 R56.2 SJ10.2 U19.5 U20.14 U20.24 U20.34 U20.44
VCC10: C91.1 C92.A C93.2 D31.A D32.A JP41.4 R61.2 R62.2 SJ11.2 U21.5 U22.14 U22.24 U22.34 U22.44
VCC11: C100.1 C101.A C102.2 D34.A D35.A JP45.4 R67.2 R68.2 SJ12.2 U23.5 U24.14 U24.24 U24.34 U24.44
VCC12: C109.1 C110.A C111.2 D37.A D38.A JP49.4 R73.2 R74.2 SJ13.2 U25.5 U26.14 U26.24 U26.34 U26.44
VCC13: C118.1 C119.A C120.2 D40.A D41.A JP53.4 R79.2 R80.2 SJ14.2 U27.5 U28.14 U28.24 U28.34 U28.44
VCC14: C127.1 C128.A C129.2 D43.A D44.A JP57.4 R85.2 R86.2 SJ15.2 U29.5 U30.14 U30.24 U30.34 U30.44
VCC15: C136.1 C137.A C138.2 D46.A D47.A JP61.4 R91.2 R92.2 SJ16.2 U31.5 U32.14 U32.24 U32.34 U32.44
VCC16: C145.1 C146.A C147.2 D49.A D50.A JP65.4 R97.2 R98.2 SJ17.2 U33.5 U34.14 U34.24 U34.34 U34.44
VCC17: C154.1 C155.A C156.2 D52.A D53.A JP69.4 R103.2 R104.2 SJ18.2 U35.5 U36.14 U36.24 U36.34 U36.44

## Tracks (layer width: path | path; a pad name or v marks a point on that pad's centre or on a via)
A0
  Top 0.203: U3.36 20.39,23.38 21.47,23.38 21.64,23.2 21.64,22.8 22.13,22.3 22.13,19.53 JP6.8
A1
  Top 0.203: U3.37 20.12,23.8 21.77,23.8 22.13,23.45 22.13,22.86 23.37,21.62 JP6.7
A2
  Top 0.203: U3.38 19.84,24.22 22.52,24.22 JP6.6
A3
  Top 0.203: 19.54,24.62 19.55,24.62 | 18.46,23.54 19.55,24.62 | 19.55,24.62 22.08,24.62 JP6.5
A8
  Top 0.203: 37.83,24.62 | 36.74,23.54 37.83,24.62 | 37.83,24.62 40.37,24.62 41.65,25.91 JP3.5
A9
  Top 0.203: U4.38 38.13,24.22 40.8,24.22 JP3.6
A10
  Top 0.203: U4.37 38.41,23.8 40.06,23.8 40.41,23.45 40.41,22.86 41.66,21.62 JP3.7
A11
  Top 0.203: U4.36 38.67,23.38 39.75,23.38 39.92,23.2 39.92,22.8 40.42,22.3 40.42,19.53 JP3.8
A14
  Top 0.203: 56.11,24.62 56.12,24.62 | 55.03,23.54 56.12,24.62 | 56.12,24.62 58.65,24.62 JP9.5
A15
  Top 0.203: U6.38 56.41,24.22 59.09,24.22 JP9.6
